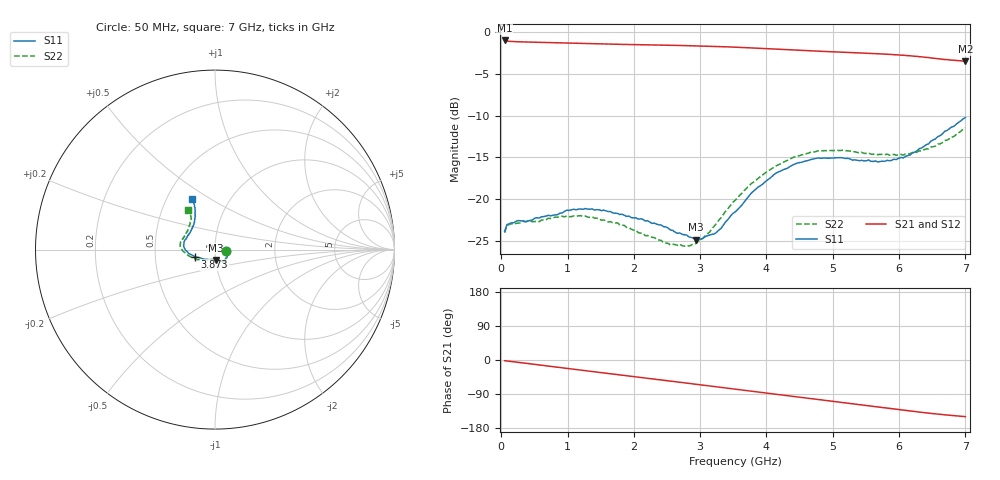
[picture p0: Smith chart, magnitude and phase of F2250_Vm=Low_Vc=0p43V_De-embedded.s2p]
! Integrated Device Technology
! Corporate Headquarters
! 6024 Silver Creek Valley Road
! San Jose, CA 95138  USA
! Phone:  1-408-284-8200
! Toll Free:  1-800-223-1366
! Webpage:  http://www.idt.com/
! Timing and RF Division
! 515 Groton Road, Suite 102
! Westford, MA 01886-6024
! Device:  F2250
! Description: Voltage Variable RF Attenuator
! Frequency:  50.0 -  6000.00 MHz
! Package:  3x3 mm Thin QFN Plastic Package: 16 pin
! Ports:  2 RF, 3 DC
!  Pin  1  = GND
!  Pin  2  = NC
!  Pin  3  = RF1  = Port 1
!  Pin  4  = NC
!  Pin  5  = GND
!  Pin  6  = GND
!  Pin  7  = GND
!  Pin  8  = GND
!  Pin  9  = NC
!  Pin 10  = RF2  = Port 2
!  Pin 11  = NC
!  Pin 12  = GND
!  Pin 13  = GND
!  Pin 14  = VCNTRL
!  Pin 15  = VDD
!  Pin 16  = VMODE
! Vcntrl:  0.430 Volts
! Vmode:  +0.000 Volts
! Vdd:  +3.30  Volts
! Current:  1.126 mA
! Data:  The device was measured on a the F2250 evaluation board which has
!  individual transmission lines to the RF pins.  Data was collected
!  using a calibrated network analyzer.  The evaluation board was
!  de-embedded using a TRL calibration technique.
!  The reference plane is the edge of the package pin.
! Misc:  SN 10
!  Action Tracker AT0258
! Date Measured:  2014-11-26
! Date:  2015-10-15  MJV
! Note:
!  Integrated Device Technology supplies this data as a sample of measured
!  data at the package pin for this product.  Your particular data for this
!  product may vary.
!  Data was taken at 25 degrees C.
!  Integrated Device Technology reserves the right to change this data at anytime.
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# GHz S dB R 50
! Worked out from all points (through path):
!   201 points, 50 MHz to 7 GHz, reference 50 ohm
!   highest |S21| = -1.01 dB at 50 MHz (marker M1); lowest = -3.5 dB at 7 GHz (marker M2)
!   group delay of S21, straight-line fit = 60 ps
!   lowest |S11| = -24.8 dB at 2.934 GHz (marker M3), VSWR 1.12, Z = 50.1 - j5.75 ohm
!   |S11| at or under -10 dB: start of sweep to end of sweep
!   |S22| runs from -25.6 to -11.5 dB; largest |S21 - S12| = 0.00037
!   S11 on the Smith chart (normalised r, x): 50 MHz: 1.14, -0.02; 3.873 GHz: 0.80, -0.07; 7 GHz: 0.67, +0.42
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0.05  -23.84 -8.6  -1.01 -1.8  -1.01 -1.8  -24.00 -9.2
0.08475  -23.04 -8.4  -1.09 -2.5  -1.09 -2.5  -23.14 -8.6
0.15425  -22.82 -10.6  -1.13 -4.0  -1.13 -4.0  -22.91 -10.3
0.57125  -22.23 -27.4  -1.24 -13.1  -1.24 -13.1  -22.67 -29.0
0.71025  -21.91 -35.1  -1.27 -16.2  -1.26 -16.2  -22.27 -36.7
1.2315  -21.19 -52.1  -1.38 -27.4  -1.38 -27.4  -22.05 -57.5
1.75275  -21.69 -58.8  -1.47 -38.5  -1.47 -38.5  -22.81 -65.5
2.37825  -23.05 -60.1  -1.56 -51.8  -1.56 -51.8  -24.87 -69.5
2.552  -23.67 -63.8  -1.59 -55.6  -1.58 -55.7  -25.47 -75.2
2.83  -24.49 -77.3  -1.64 -61.7  -1.63 -61.7  -25.59 -93.1
2.93425  -24.84 -85.4  -1.66 -64.1  -1.65 -64.0  -25.29 -101.2
3.21225  -24.14 -113.7  -1.72 -70.2  -1.72 -70.2  -23.20 -125.6
3.525  -21.53 -141.9  -1.81 -77.2  -1.82 -77.2  -20.13 -144.6
3.8725  -18.54 -160.0  -1.94 -84.8  -1.94 -84.8  -17.51 -160.2
4.1505  -16.83 -170.3  -2.06 -90.9  -2.06 -90.9  -15.98 -170.3
4.4285  -15.79 -178.2  -2.16 -96.9  -2.16 -96.9  -14.92 -177.6
4.7065  -15.18 174.8  -2.27 -102.9  -2.27 -102.9  -14.36 176.3
5.15825  -15.06 164.0  -2.43 -112.7  -2.43 -112.7  -14.12 167.0
5.85325  -15.39 140.7  -2.67 -127.6  -2.67 -127.6  -14.72 151.7
6.166  -14.71 129.4  -2.84 -134.4  -2.84 -134.4  -14.55 142.8
6.444  -13.38 120.7  -3.05 -140.2  -3.05 -140.2  -13.97 133.4
7  -10.22 114.0  -3.49 -149.5  -3.49 -149.5  -11.47 123.9
